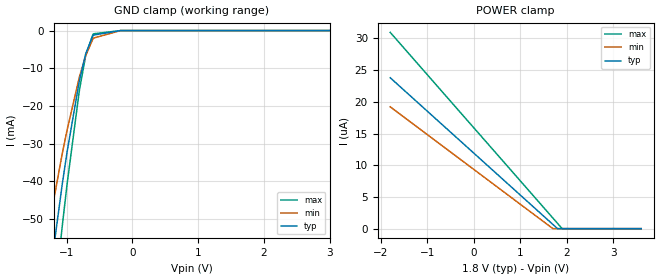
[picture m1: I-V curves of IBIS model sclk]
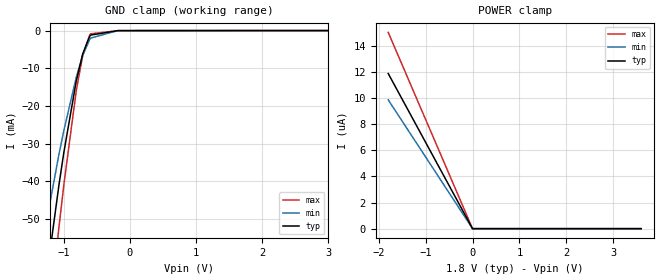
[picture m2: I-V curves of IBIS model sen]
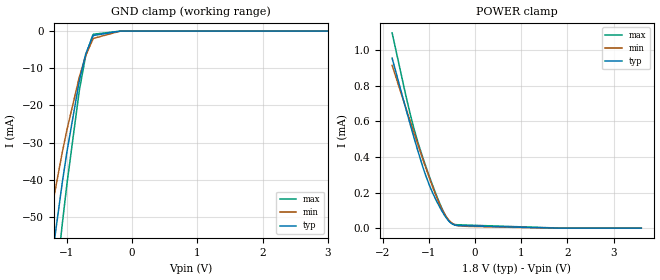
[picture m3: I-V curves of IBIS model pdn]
|Texas Instruments Incorporated
| Quad 14-bit 25 - 125 Msps Analog to Digital Converter
| Marketing part#   Digital Voltage Range   Package-type   #pins
| ADC3244IRTQT   1.7V-1.9V   QFN   48
| ADC3244IRTQR   1.7V-1.9V   QFN   48
[IBIS Ver]   4.1
[File name]   adc3244.ibs
[File Rev]   1.0
[Date]   5/8/2014
[Source]
| Texas Instruments Incorporated.
| Analog-eLab Design Center, HPA
| 12500 TI Blvd
| Dallas, TX -75243
[Notes]   Revision History:
| Rev 1.0: 5/8/2014
| - Initial version of the model
| - Model generated from simulations in TISPICE
| - Model matched to SPICE simulation
| - C_comp although listed in numerical order of value are
|   obtained from varying PVT conditions. For PVT conditions for
|   each specific value refer the buffer description under
|   respective [Model]. IBIS model user is responsible for using
|   appropriate C_comp to simulate for Signal Integrity.
| - This is a relative part of ADC3444.
|* EXCEPTION:   *
|* - For model sclk and reset, There will be a leakage current in the   *
|*   POWER clamp I-V Table because of two resistors(R1 & R2) connected  *
|*   to Pad.   *
|* - For model sen, There will be a leakage current in GND clamp I-V   *
|*   Table because of two resistors network(R1 & R2) connected to Pad.  *
|* - For model pdn, There will be a leakage current in the POWER Clamp  *
|*   I-V Table because of Transistor MP3 connected to Pad.   *
|* - For model clk and sysref, There will be a leakage current in both  *
|*   POWER and GND clamp I-V Table because of the resistor network (R6) *
|*   connected to Pad.   *
|* - For lvds, Pullup and Pulldown will not pass through zero due to   *
|*   driver switch(MP1 and MN1) arrangement.   *
[Disclaimer]
| This model is designed as an aid for customers of Texas Instruments.
| TI and its licensors and suppliers make no warranties, either expressed
| or implied, with respect to this  model, including the warranties of
| merchantability or fitness for a particular purpose. The model is
| provided solely on an "as is" basis. The entire risk as to its quality
| and performance is with the customer.
[Copyright]
(C) Copyright 2014 Texas Instruments Incorporated.All rights reserved.
|   ADC3244RGZ
[Component]   ADC3244RGZ
[Manufacturer]   TI
[Package]   |48 QFN   -  RGZ package
|   typ   min   max
R_pkg   0.157452   0.0729   0.20281
L_pkg   1.516274nH   1.01014nH   1.9466nH
C_pkg   0.19146pF   0.16682pF   0.23003pF
[Pin]  signal_name   model_name   R_pin   L_pin   C_pin
1   GND   gnd   0.00663   0.18384nH   1.9099pF
2   DVDD   power   0.07534   1.09053nH   0.2151pF
3   GND   gnd   0.06837   0.957nH   0.20468pF
4   DVDD   power   0.06726   0.93599nH   0.20074pF
5   GND   gnd   0.06469   0.88707nH   0.19989pF
6   AVDD   power   0.06554   0.90138nH   0.1967pF
7   AVDD   power   0.06837   0.95269nH   0.21409pF
8   AVDD   power   0.06595   0.90873nH   0.20952pF
9   AVDD   power   0.06573   0.9049nH   0.21995pF
10   INAP   nc   0.06901   0.96464nH   0.21975pF
11   INAM   nc   0.07632   1.10205nH   0.24294pF
12   AVDD   power   0.08327   1.27847nH   0.21691pF
13   SCLK   sclk   0.20269   1.9466nH   0.21472pF
14   SDATA   sclk   0.18535   1.76583nH   0.21381pF
15   SEN   sen   0.17001   1.60989nH   0.19981pF
16   SDOUT   sdout   0.15736   1.48194nH   0.19207pF
17   AVDD   power   0.07498   1.05995nH   0.2306pF
18   CLKP   clk   0.0729   1.01189nH   0.22858pF
19   CLKM   clk   0.0729   1.01014nH   0.22852pF
20   AVDD   power   0.07498   1.05512nH   0.23047pF
21   RESET   reset   0.15736   1.47705nH   0.19244pF
22   SYSREFP   sysref   0.17343   1.63789nH   0.20211pF
23   SYSREFM   sysref   0.19899   1.89583nH   0.23003pF
24   VCM   nc   0.11058   1.82307nH   0.28543pF
25   AVDD   power   0.08327   1.27502nH   0.21666pF
26   INBM   nc   0.07632   1.10569nH   0.24246pF
27   INBP   nc   0.06901   0.96491nH   0.21926pF
28   AVDD   power   0.06573   0.90256nH   0.21442pF
29   AVDD   power   0.06595   0.90666nH   0.20412pF
30   AVDD   power   0.06837   0.95256nH   0.22199pF
31   PDN   pdn   0.1311   1.213nH   0.16954pF
32   GND   gnd   0.06472   0.883nH   0.19776pF
33   DVDD   power   0.0662   0.90887nH   0.19734pF
34   GND   gnd   0.1331   1.2331nH   0.16354pF
35   DVDD   power   0.07534   1.07953nH   0.21016pF
36   GND   gnd   0.15461   1.45411nH   0.15757pF
37   DB1P   lvds   0.20281   1.9394nH   0.1957pF
38   DB1M   lvds   0.17661   1.67053nH   0.19455pF
39   DB0P   lvds   0.16373   1.54069nH   0.18306pF
40   DB0M   lvds   0.14802   1.38444nH   0.16975pF
41   FCLKP   lvds   0.15385   1.44211nH   0.17266pF
42   FCLKM   lvds   0.14361   1.3413nH   0.16794pF
43   DCLKP   lvds   0.14289   1.33508nH   0.16737pF
44   DCLKM   lvds   0.15089   1.4166nH   0.1705pF
45   DA1P   lvds   0.14443   1.35102nH   0.16682pF
46   DA1M   lvds   0.15618   1.47019nH   0.1773pF
47   DA0P   lvds   0.16735   1.58371nH   0.18716pF
48   DA0M   lvds   0.19148   1.8329nH   0.18768pF
[Diff_pin]   inv_pin   vdiff   tdelay_typ   tdelay_min   tdelay_max
18   19   200mV   NA   NA   NA
22   23   200mV   NA   NA   NA
37   38   NA   0   0   0
39   40   NA   0   0   0
41   42   NA   0   0   0
43   44   NA   0   0   0
45   46   NA   0   0   0
47   48   NA   0   0   0
| Models and submodels in the file (8): sclk (Input), sen (Input), pdn (Input), reset (Input), clk (Input), sysref (Input), sdout (Output), lvds (Output)
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|   sclk Model
[Model]   sclk
Model_type   Input
Vinl = 0.4
Vinh = 1.2
|   typ   min   max
|   (nom PVT)   (fast PVT)   (slow PVT)
C_comp   1.286e-12   1.247e-12   1.328e-12
| Where nom  PVT is Nominal Process, 1.8V, 27C
|   Fast PVT is Strong Process,  1.9V, -40C
|   Slow PVT is Weak Process,   1.7V, 125C
[Voltage Range]   1.8   1.7   1.9
|Junction Temperature
[Temperature Range]   27   125   -40
[Power Clamp Reference]   1.8   1.7   1.9
[GND Clamp Reference]   0   0   0
[GND Clamp]
|   Voltage   I(typ)   I(min)   I(max)
-1.8V     -793.1mA   -162.8mA   -1.722A
-1.364V   -79.24mA   -60.76mA   -100.9mA
-1.069V   -40.88mA   -32.75mA   -52.04mA
-994.2mV  -32.22mA   -26.42mA   -40.77mA
-811.8mV  -13.8mA    -12.68mA   -16.5mA
-802.1mV  -12.96mA   -12.04mA   -15.41mA
-710.3mV  -6.172mA   -6.645mA   -6.588mA
-603mV    -1.45mA    -2.287mA   -1.097mA
-592.2mV  -1.193mA   -1.991mA   -857.2uA
-180mV    -1.194uA   -1.237uA   -1.505uA
3.6V      0A         0A         0A
[POWER Clamp]
|   Voltage   I(typ)   I(min)   I(max)
-1.8V     23.79uA    19.2uA     30.94uA
1.699V    670nA      0A         1.684uA
1.798V    11.89nA    0A         851.2nA
1.899V    0A         0A         0A
3.6V      0A         0A         0A
|   sen Model
[Model]   sen
Model_type   Input
Vinl = 0.4
Vinh = 1.2
|   typ   min   max
|   (nom PVT)   (fast PVT)   (slow PVT)
C_comp   1.286e-12   1.247e-12   1.328e-12
| Where nom  PVT is Nominal Process, 1.8V, 27C
|   Fast PVT is Strong Process,  1.9V, -40C
|   Slow PVT is Weak Process,   1.7V, 125C
[Voltage Range]   1.8   1.7   1.9
|Junction Temperature
[Temperature Range]   27   125   -40
[Power Clamp Reference]   1.8   1.7   1.9
[GND Clamp Reference]   0   0   0
[GND Clamp]
|   Voltage   I(typ)   I(min)   I(max)
-1.8V     -793.1mA   -162.8mA   -1.722A
-1.364V   -79.25mA   -60.76mA   -100.9mA
-1.069V   -40.88mA   -32.76mA   -52.05mA
-994.2mV  -32.23mA   -26.42mA   -40.77mA
-811.8mV  -13.8mA    -12.68mA   -16.51mA
-802.1mV  -12.97mA   -12.04mA   -15.42mA
-710.3mV  -6.178mA   -6.65mA    -6.597mA
-604.9mV  -1.508mA   -2.349mA   -1.156mA
-592.2mV  -1.202mA   -1.998mA   -870.2uA
-180mV    -13.09uA   -10.56uA   -17.39uA
3.6V      0A         0A         0A
[POWER Clamp]
|   Voltage   I(typ)   I(min)   I(max)
-1.8V     11.89uA    9.877uA    15.05uA
-1.4mV    0A         0A         11.72nA
-700uV    0A         0A         0A
3.6V      0A         0A         0A
|   pdn Model
[Model]   pdn
Model_type   Input
Vinl = 0.4
Vinh = 1.2
|   typ   min   max
|   (nom PVT)   (fast PVT)   (slow PVT)
C_comp   1.247e-12   1.193e-12   1.292e-12
| Where nom  PVT is Nominal Process, 1.8V, 27C
|   Fast PVT is Strong Process,  1.9V, -40C
|   Slow PVT is Weak Process,   1.7V, 125C
[Voltage Range]   1.8   1.7   1.9
|Junction Temperature
[Temperature Range]   27   125   -40
[Power Clamp Reference]   1.8   1.7   1.9
[GND Clamp Reference]   0   0   0
[GND Clamp]
|   Voltage   I(typ)   I(min)   I(max)
-1.8V     -792mA     -161.9mA   -1.721A
-1.368V   -79.06mA   -60.56mA   -100.7mA
-1.07V    -40.73mA   -32.6mA    -51.86mA
-999.3mV  -32.49mA   -26.57mA   -41.14mA
-813.6mV  -13.81mA   -12.66mA   -16.54mA
-803.8mV  -12.97mA   -12.02mA   -15.44mA
-712mV    -6.205mA   -6.654mA   -6.646mA
-604.9mV  -1.481mA   -2.313mA   -1.131mA
-592.2mV  -1.179mA   -1.966mA   -848.3uA
-180mV    -1.184uA   -1.221uA   -1.493uA
3.6V      0A         0A         0A
[POWER Clamp]
|   Voltage   I(typ)   I(min)   I(max)
-1.8V     954.5uA    914.1uA    1.097mA
-1.469V   639.2uA    648.2uA    707uA
-1.323V   505.6uA    533.1uA    555.5uA
-1.24V    431.7uA    467.9uA    480.2uA
-1.073V   296.6uA    340.8uA    349uA
-928.8mV  202.3uA    236.3uA    244.9uA
-718.2mV  95.06uA    104.9uA    109.5uA
-549mV    33.87uA    39.06uA    34.98uA
-432mV    16.76uA    17.65uA    20.17uA
-180mV    12.95uA    10.23uA    17.22uA
1.899V    0A         0A         0A
3.6V      0A         0A         0A
